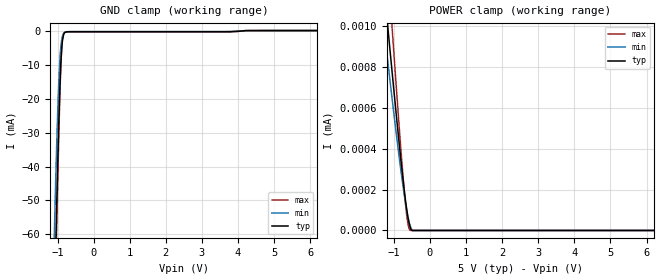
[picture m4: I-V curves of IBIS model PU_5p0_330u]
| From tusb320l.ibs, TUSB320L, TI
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|   Model
[Model]   PU_5p0_330u
Model_type   Input
Vinl = 1.5
Vinh = 3.5
|   typ   min   max
C_comp   0.475pF   0.451pF   0.489pF
[Voltage Range]   5   4.999   5.001
[Temperature Range]   27   105   -40
[Power Clamp Reference]   5   4.999   5.001
[GND Clamp Reference]   0   0   0
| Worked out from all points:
|   GND clamp passes 1 mA (typ) near -0.82 V on its own axis
[GND Clamp]
|   Voltage   I(typ)   I(min)   I(max)
-5V       -2.345A    -2.242A    -2.422A
-1.085V   -81.6mA    -58.9mA    -91.17mA
-1.04V    -59.78mA   -40.22mA   -67.58mA
-1.025V   -52.82mA   -34.5mA    -59.96mA
-995mV    -39.55mA   -24.07mA   -45.25mA
-965mV    -27.46mA   -15.37mA   -31.53mA
-935mV    -17.1mA    -8.82mA    -19.39mA
-905mV    -9.17mA    -4.562mA   -9.789mA
-890mV    -6.305mA   -3.195mA   -6.319mA
-860mV    -2.706mA   -1.559mA   -2.252mA
-800mV    -603.3uA   -511.5uA   -496uA
10V       0A         0A         0A
[POWER Clamp]
|   Voltage   I(typ)   I(min)   I(max)
-5V       8.523uA    1.593A     11.61uA
-1.91V    2.427uA    87.48uA    3.265uA
-1.25V    1.158uA    959.6nA    1.521uA
-1.145V   960.8nA    797.1nA    1.249uA
-1.04V    766.4nA    637.3nA    979.9nA
-830mV    392.3nA    332.2nA    461.8nA
-695mV    176.2nA    158.2nA    166.7nA
-650mV    114.5nA    108.4nA    88.13nA
-605mV    62.54nA    65.62nA    31.31nA
-530mV    8.341nA    15.64nA    0A
-485mV    0A         0A         0A
10V       0A         0A         0A
